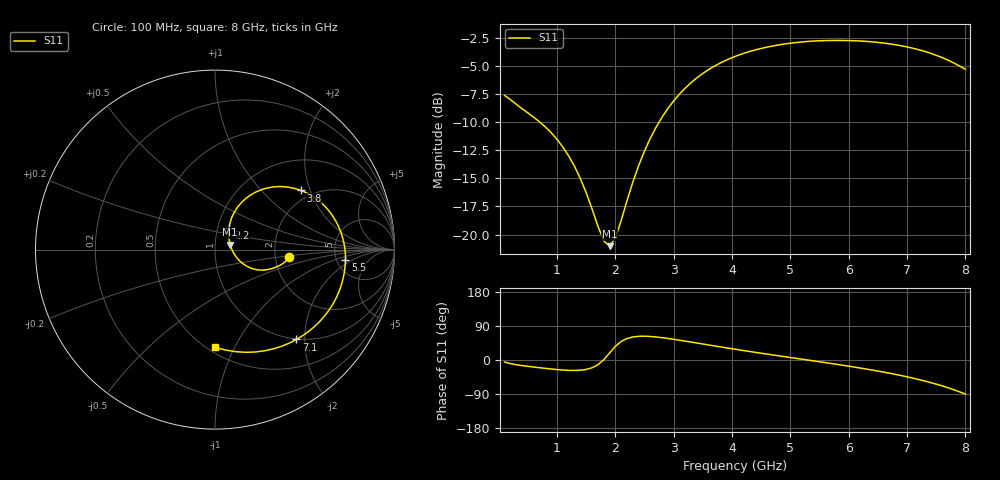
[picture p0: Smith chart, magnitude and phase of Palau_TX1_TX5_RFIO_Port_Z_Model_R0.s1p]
! Created Fri Jul 10 09:34:16 2020
! Palau TX1/TX5 RFIO Port Impedance Model.
! Revision		: R0.
! Impedance Mode 	: Balanced Differential-Mode.
! Impedance Format 	: Series Equivalent Differential Impedance (SEDZ).
# hz S ma R 50
! 1 Port Network Data from SP1.SP block
! freq  magS11  angS11
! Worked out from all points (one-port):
!   80 points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, 100 MHz to 8 GHz, reference 50 ohm
!   lowest |S11| = -21.0 dB at 1.9 GHz (marker M1), VSWR 1.19, Z = 59.1 + j3.37 ohm
!   |S11| at or under -10 dB: 707.2 MHz to 2.748 GHz (2.04 GHz wide, 118 % of centre)
!   S11 on the Smith chart (normalised r, x): 100 MHz: 2.40, -0.23; 2.2 GHz: 1.13, +0.27; 3.8 GHz: 1.74, +1.73; 5.5 GHz: 5.99, -1.53; 7.1 GHz: 0.99, -1.82; 8 GHz: 0.54, -0.84
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1e8  0.4164 -5.4
3e8  0.3802 -12.5
5e8  0.3478 -16.7
8e8  0.3012 -22.1
1.1e9  0.245 -26.5
1.4e9  0.1772 -26.9
1.8e9  0.09368 0.8
1.9e9  0.08873 18.6
2e9  0.09677 36.3
2.1e9  0.1158 49.1
2.2e9  0.1418 56.8
2.4e9  0.2034 62.5
2.6e9  0.2689 62.0
2.8e9  0.3334 58.9
3.1e9  0.4226 52.2
3.4e9  0.4994 44.7
3.8e9  0.5811 34.6
4.1e9  0.628 27.3
4.6e9  0.6833 15.6
5.1e9  0.7162 4.4
5.5e9  0.7293 -4.7
6.1e9  0.7294 -18.7
6.6e9  0.7123 -32.0
7.1e9  0.6755 -47.9
7.4e9  0.6419 -59.4
7.6e9  0.6138 -68.3
7.8e9  0.5809 -78.4
8e9  0.5447 -90.1
